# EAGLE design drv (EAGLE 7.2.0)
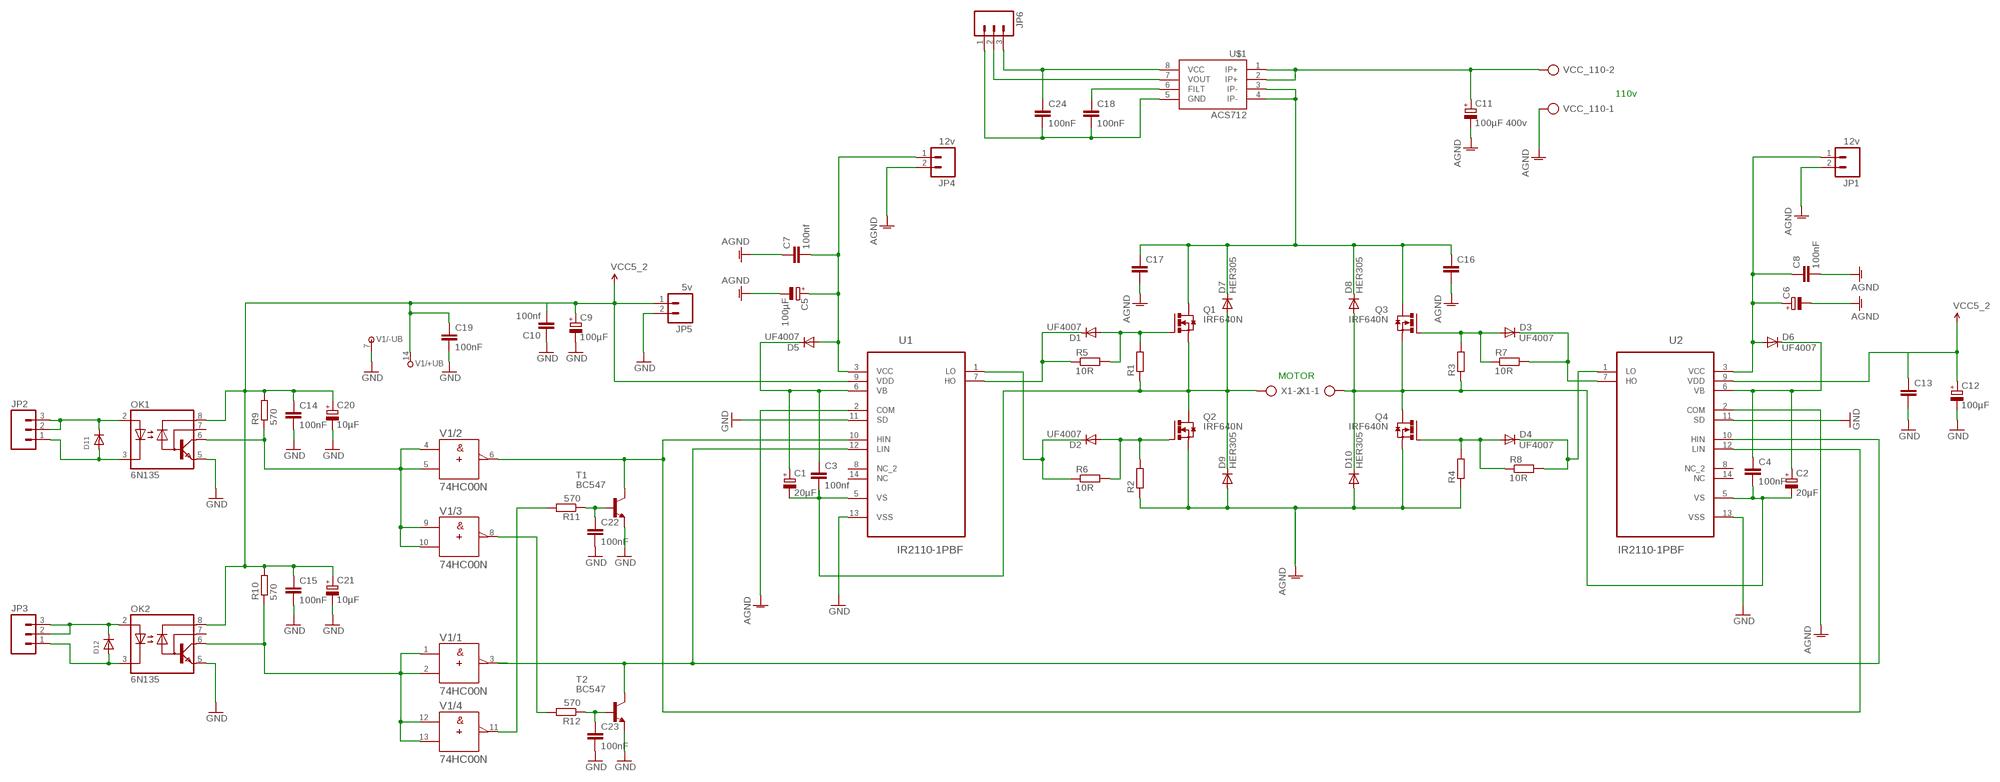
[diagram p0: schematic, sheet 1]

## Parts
C1  20µF  CPOL-EUE2,5-6E  [E2,5-6E]
C2  20µF  CPOL-EUE2,5-6E  [E2,5-6E]
C3  100nf  C-EUC0805  [C0805]
C4  100nF  C-EUC0504  [C0504]
C5  100µF  CPOL-EUE2-5  [E2-5]
C6  CPOL-EUE2-5  [E2-5]
C7  100nf  C-EUC1310  [C1310]
C8  100nF  C-EUC0805  [C0805]
C9  100µF  CPOL-EUE2-5  [E2-5]
C10  100nf  C-EUC0805  [C0805]
C11  100µF 400v  CPOL-EUE10-25  [EB25D]
C12  100µF  CPOL-EUE2-5  [E2-5]
C13  C-EUC0805  [C0805]
C14  100nF  C-EUC0805  [C0805]
C15  100nF  C-EUC0805  [C0805]
C16  C5/3  [C5B3]
C17  C5/3  [C5B3]
C18  100nF  C-EUC0805  [C0805]
C19  100nF  C-EUC0805  [C0805]
C20  10µF  CPOL-EUE2-5  [E2-5]
C21  10µF  CPOL-EUE2-5  [E2-5]
C22  100nF  C-EUC0402  [C0402]
C23  100nF  C-EUC0402  [C0402]
C24  100nF  C-EUC0805  [C0805]
D1  UF4007  DIODE  [DIODE-1N4001-KIT]
D2  UF4007  DIODE  [DIODE-1N4001-KIT]
D3  UF4007  DIODE  [DIODE-1N4001-KIT]
D4  UF4007  DIODE  [DIODE-1N4001-KIT]
D5  UF4007  DIODE  [DIODE-1N4001-KIT]
D6  UF4007  DIODE  [DIODE-1N4001-KIT]
D7  HER305  1N5624  [DO201-15]
D8  HER305  1N5624  [DO201-15]
D9  HER305  1N5624  [DO201-15]
D10  HER305  1N5624  [DO201-15]
D11  DIODEDO-1N4148  [DO-1N4148]
D12  DIODEDO-1N4148  [DO-1N4148]
JP1  12v  M02JST-PTH-VERT  [JST-2-PTH-VERT]
JP2  M03LOCK  [1X03_LOCK]
JP3  M03LOCK  [1X03_LOCK]
JP4  12v  M02JST-PTH-VERT  [JST-2-PTH-VERT]
JP5  5v  M02JST-PTH-VERT  [JST-2-PTH-VERT]
JP6  M03LOCK  [1X03_LOCK]
OK1  6N135  [DIL08]
OK2  6N135  [DIL08]
Q1  IRF640N  IRF3704L-V  [TO262-V]
Q2  IRF640N  IRF3704L-V  [TO262-V]
Q3  IRF640N  IRF3704L-V  [TO262-V]
Q4  IRF640N  IRF3704L-V  [TO262-V]
R1  R-EU_0207/12  [0207/12]
R2  R-EU_0207/12  [0207/12]
R3  R-EU_0207/12  [0207/12]
R4  R-EU_0207/12  [0207/12]
R5  10R  R-EU_0207/12  [0207/12]
R6  10R  R-EU_0207/12  [0207/12]
R7  10R  R-EU_0207/12  [0207/12]
R8  10R  R-EU_0207/12  [0207/12]
R9  570  R-EU_R0805  [R0805]
R10  570  R-EU_R0805  [R0805]
R11  570  R-EU_0204/7  [0204/7]
R12  570  R-EU_0204/7  [0204/7]
T1  BC547  [TO92]
T2  BC547  [TO92]
U1  IR2110-1PBF  [DIP254P762X533-14]
U2  IR2110-1PBF  [DIP254P762X533-14]
U$1  ACS712  [SO08]
V1  74HC00N  [DIL14]
VCC_110  AK300/2  [AK300/2]
X1  AK300/2  [AK300/2]

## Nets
AGND: C5.- C6.- C7.1 C8.2 C11.- C16.2 C17.2 D9.A D10.A JP1.2 JP4.2 Q2.3(S) Q4.3(S) R2.1 R4.1 U1.2(COM) U2.2(COM) VCC_110.1
GND: C9.- C10.1 C12.- C13.2 C14.2 C15.2 C19.2 C20.- C21.- C22.2 C23.2 JP5.2 OK1.5(GND) OK2.5(GND) T1.1(E) T2.1(E) U1.11(SD) U1.13(VSS) U2.11(SD) U2.13(VSS) V1.7(/-UB:-UB)
H_PVR1: C11.+ U$1.1(IP+) U$1.2(IP+) VCC_110.2
N$1: D1.A Q1.1(G) R1.2 R5.2
N$2: C18.1 U$1.6(FILT)
N$3: D11.C JP2.2 JP2.3 OK1.2(A)
N$4: D2.A Q2.1(G) R2.2 R6.2
N$5: D1.C R5.1 U1.7(HO)
N$6: D11.A JP2.1 OK1.3(C)
N$7: D2.C R6.1 U1.1(LO)
N$8: R11.2 V1.11(/4:Y)
N$9: D3.A Q3.1(G) R3.2 R7.1
N$10: D3.C R7.2 U2.7(HO)
N$11: D4.C R8.2 U2.1(LO)
N$12: D12.A JP3.1 OK2.3(C)
N$14: D4.A Q4.1(G) R4.2 R8.1
N$15: C1.+ C3.1 D5.C U1.6(VB)
N$16: T1.3(C) U1.10(HIN) U2.12(LIN) V1.6(/2:Y)
N$17: C2.+ C4.1 D6.C U2.6(VB)
N$18: C18.2 C24.2 JP6.1 U$1.5(GND)
N$19: T2.3(C) U1.12(LIN) U2.10(HIN) V1.3(/1:Y)
N$20: R12.2 V1.8(/3:Y)
N$21: OK1.6(VO) R9.1 V1.4(/2:A) V1.5(/2:B) V1.9(/3:A) V1.10(/3:B)
N$22: C22.1 R11.1 T1.2(B)
N$23: C23.1 R12.1 T2.2(B)
N$24: C24.1 JP6.3 U$1.8(VCC)
N$25: OK2.6(VO) R10.1 V1.1(/1:A) V1.2(/1:B) V1.12(/4:A) V1.13(/4:B)
N$26: D12.C JP3.2 JP3.3 OK2.2(A)
N$28: JP6.2 U$1.7(VOUT)
OUT1: C2.- C4.2 D8.A D10.C Q3.3(S) Q4.2(D) R3.1 U2.5(VS) X1.1
OUT2: C1.- C3.2 D7.A D9.C Q1.3(S) Q2.2(D) R1.1 U1.5(VS) X1.2
VCC: C9.+ C10.2 C12.+ C13.1 C14.1 C15.1 C19.1 C20.+ C21.+ JP5.1 OK1.8(VCC) OK2.8(VCC) R9.2 R10.2 U1.9(VDD) U2.9(VDD) V1.14(/+UB:+UB) ; supply symbol labelled VCC5_2
VCC_12_1: C5.+ C7.2 D5.A JP4.1 U1.3(VCC)
VCC_12_2: C6.+ C8.1 D6.A JP1.1 U2.3(VCC)
VCC_110: C16.1 C17.1 D7.C D8.C Q1.2(D) Q3.2(D) U$1.3(IP-) U$1.4(IP-)
Unconnected: OK1.7(VB) OK2.7(VB) U1.8(NC_2) U1.14(NC) U2.8(NC_2) U2.14(NC)

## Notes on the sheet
- 110v
- MOTOR

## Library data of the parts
C1 C2 C5 C6 C9 C11 C12 C20 C21 = rcl:CPOL-EU: POLARIZED CAPACITOR, European symbol
C3 C4 C7 C8 C10 C13-C15 C18 C19 C22-C24 = rcl:C-EU: CAPACITOR, European symbol
C16 C17 = capacitor-wima:C: CAPACITOR
D1-D6 = SparkFun-DiscreteSemi:DIODE: Diode
D7-D10 = diode:1N5624: DIODE
D11 D12 = adafruit:DIODE: Diode
JP1 JP4 JP5 = SparkFun-Connectors:M02: Standard 2-pin 0.1" header. Use with
JP2 JP3 JP6 = SparkFun-Connectors:M03: Header 3 Standard 3-pin 0.1" header. Use with straight break away headers (SKU : PRT-00116), right angle break away headers (PRT-00553), swiss pins (PRT-00743), machine pins (PRT-00117), and female headers (PRT-00115). Molex polarized connector foot print use with SKU : PRT-08232 with associated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
OK1 OK2 = optocoupler:6N135: MOTOROLA OPTO COUPLER; MF: FAIRCHILD SEMICONDUCTOR; MPN: 6N135; OC_FARNELL: 1021342; OC_NEWARK: 58K9658
Q1-Q4 = transistor-power:IRF3704: SMPS MOSFET HEXFET® Power MOSFET Source: http://www.irf.com/product-info/datasheets/data/irf3704.pdf
R1-R12 = rcl:R-EU_: RESISTOR, European symbol
T1 T2 = transistor:BC547: NPN TRANSISTOR
U1 U2 = International_Rectifier_By_element14_Batch_1:IR2110-1PBF: HIGH AND LOW SIDE DRIVER; MPN: IR2110-1PBF; OC_FARNELL: 1374799; OC_NEWARK: 19K8414; PACKAGE: PDIP-14; SUPPLIER: INTERNATIONAL RECTIFIER
U$1 = SparkFun-AnalogIC:ACS712: Hall-effect-based isolated linear current sensor
V1 = 74ttl-din:74*00: Quad 2-input NAND gate
VCC_110 X1 = con-ptr500:AK300/2: CONNECTOR; OC_FARNELL: unknown; OC_NEWARK: unknown

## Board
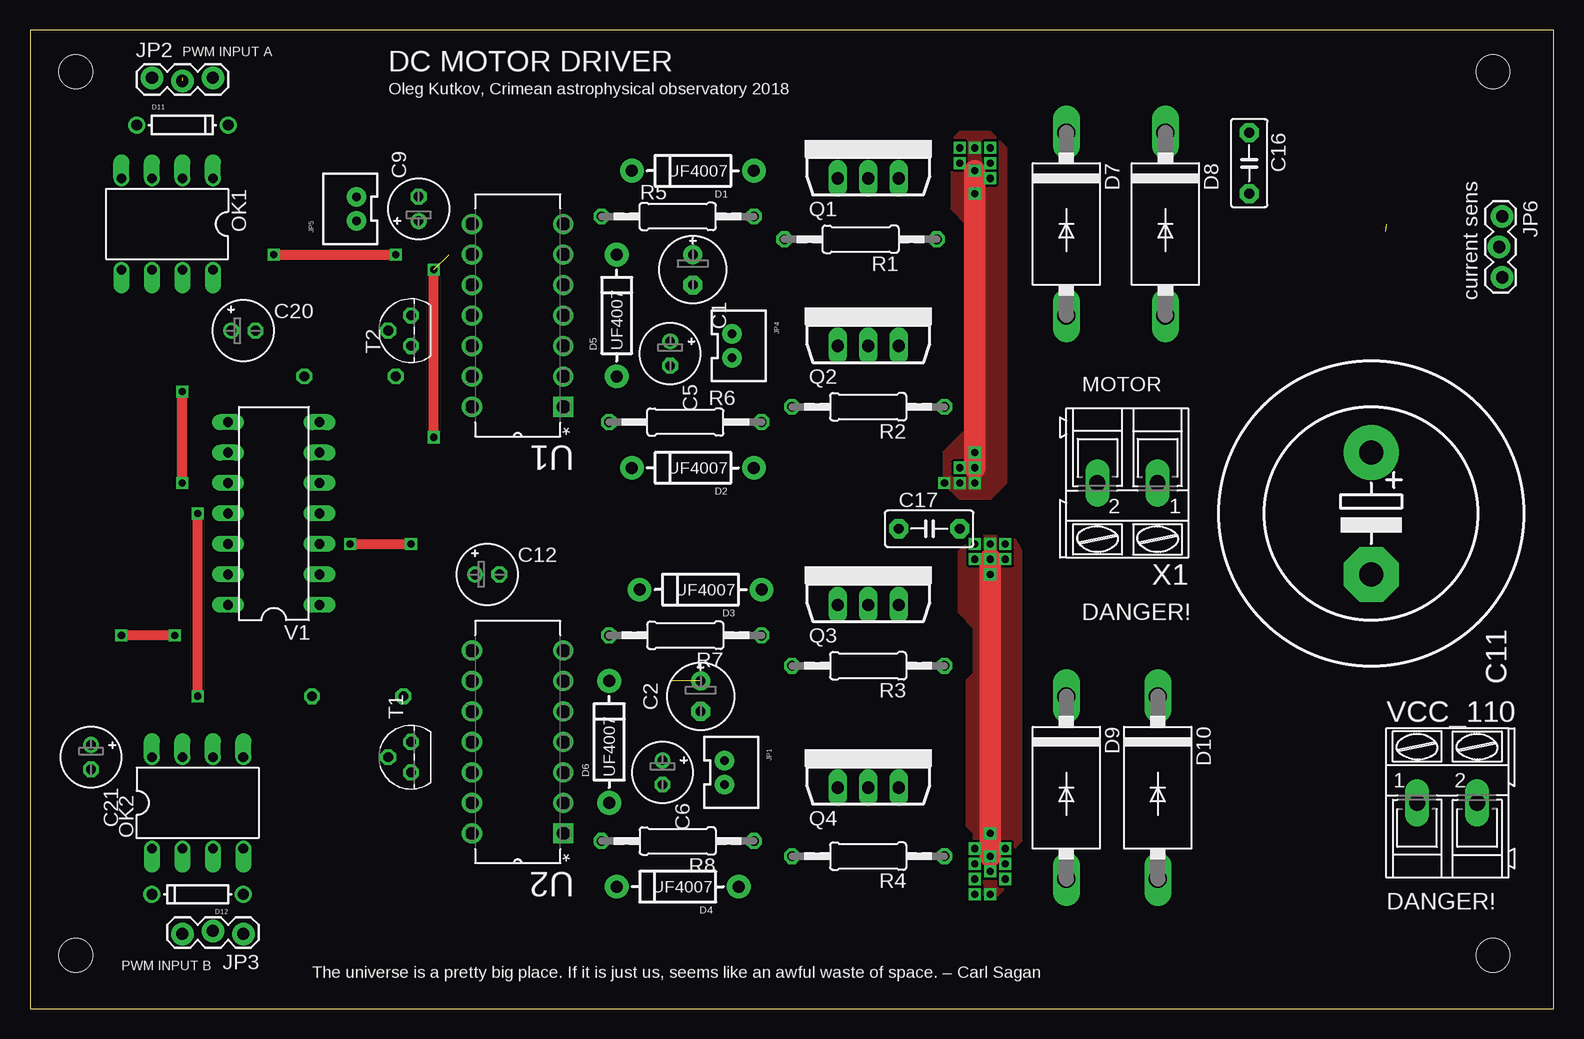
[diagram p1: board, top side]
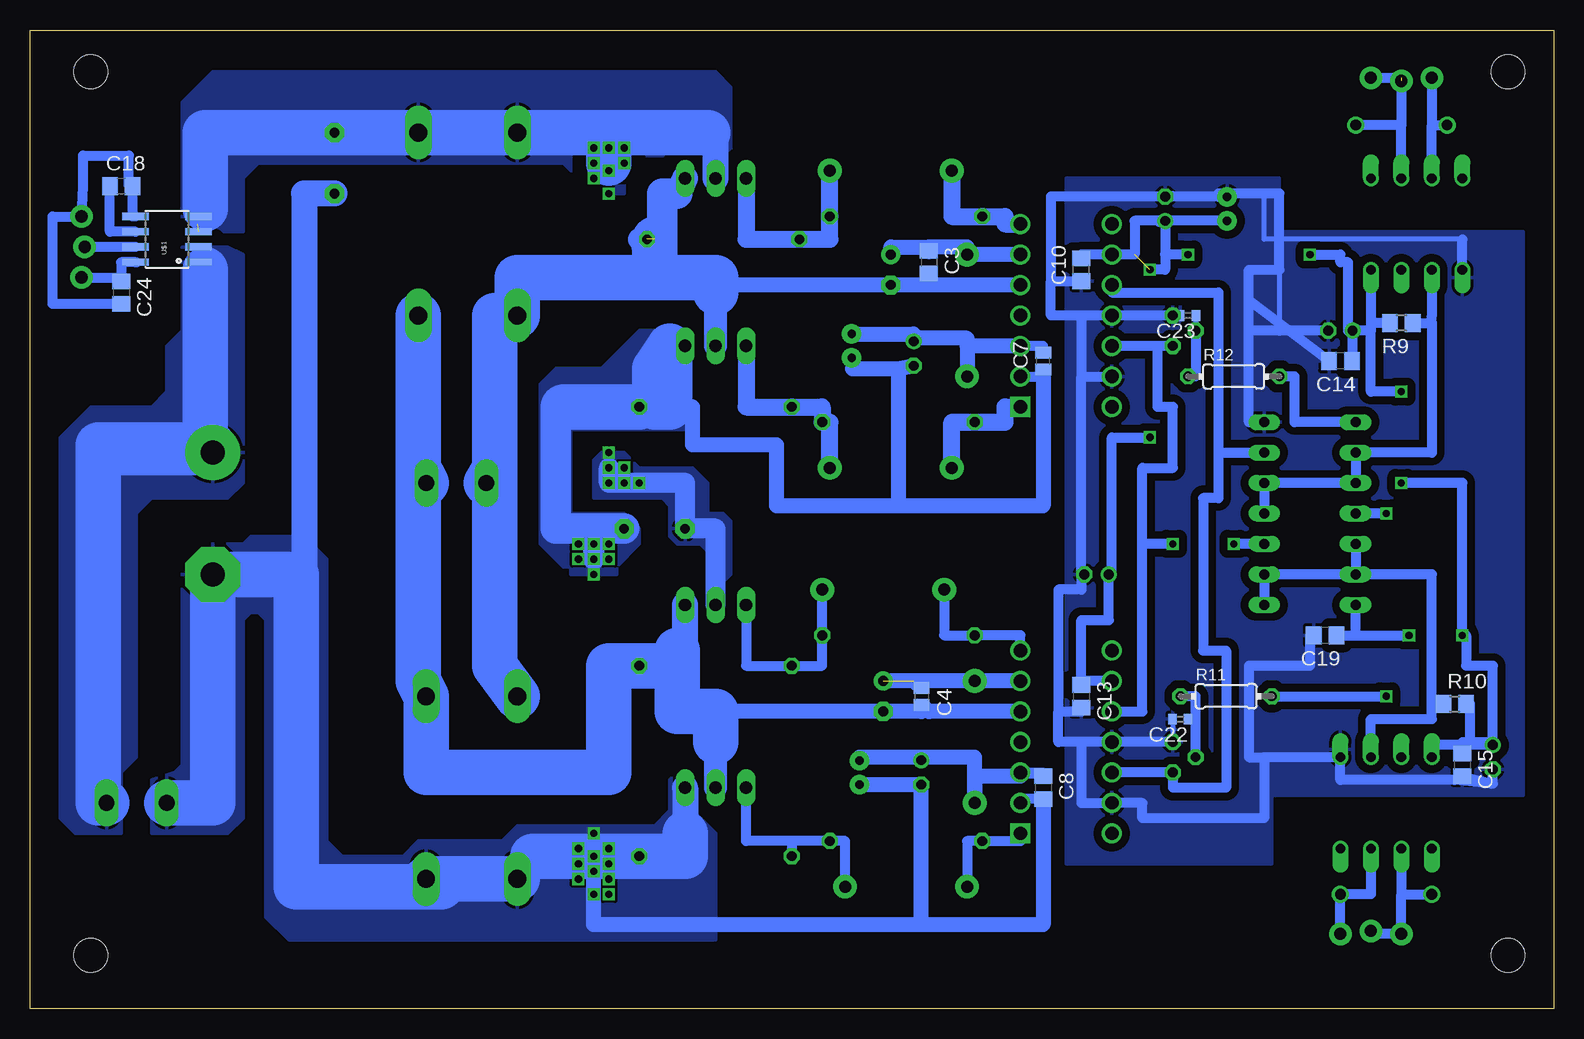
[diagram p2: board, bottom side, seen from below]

Size 126.98 x 81.58 mm. Coordinates in mm from the lower left corner, seen from the top.
Outline: 0,0 126.98,0 126.98,81.58 0,81.58 0,0
Copper layers (1*16): Top 0.035mm / dielectric 1.5mm / Bottom 0.035mm
Design rules "default": minimum track width 10mil, minimum drill 24mil, track to track 8mil, track to pad 8mil, pad to pad 8mil, via to via 8mil, smd to smd 8mil, copper to edge 40mil, drill to drill 8mil, minimum pad ring 10mil, minimum via ring 8mil, stop-mask expansion 4mil, vias tented up to drill 0mil, thermal gap 10mil
Holes 2.8 mm at 3.81,78.11 121.92,78.11 121.92,4.44 3.81,4.44

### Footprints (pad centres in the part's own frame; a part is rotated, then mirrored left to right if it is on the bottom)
E2,5-6E = drill 0.813 pad 1.575: + -1.27,0 | drill 0.813 pad 1.575 octagon: - 1.27,0
C0805 = smd 1.3 x 1.5: 1 -0.95,0; 2 0.95,0
C0504 = smd 1 x 1.3: 1 -0.7,0; 2 0.7,0
E2-5 = drill 0.813 pad 1.27: + -1.016,0 | drill 0.813 pad 1.27 octagon: - 1.016,0
C1310 = smd 1 x 1.3: 1 -0.7,0; 2 0.7,0
EB25D = drill 2.007 pad 4.597: + -5.08,0 | drill 2.007 pad 4.597 octagon: - 5.08,0
C5B3 = drill 0.813 pad 1.6 octagon: 1 -2.54,0; 2 2.54,0
C0402 = smd 0.7 x 0.9: 1 -0.65,0; 2 0.65,0
DIODE-1N4001-KIT = drill 1 pad 1.981: A -5.08,0; C 5.08,0
DO201-15 = drill 1.499 long: A 7.62,0; C -7.62,0
DO-1N4148 = drill 0.9: A -3.81,0; C 3.81,0
JST-2-PTH-VERT = drill 0.7 pad 1.626: 1 -1,-0.55; 2 1,-0.55
1X03_LOCK = drill 1.016 pad 1.88: 1 0,0.127; 2 2.54,-0.127; 3 5.08,0.127
DIL08 = drill 0.813 offset: 1 -3.81,-3.81; 2 -1.27,-3.81; 3 1.27,-3.81; 4 3.81,-3.81; 5 3.81,3.81; 6 1.27,3.81; 7 -1.27,3.81; 8 -3.81,3.81
TO262-V = drill 1.016 long: 1 -2.54,0; 2 0,0; 3 2.54,0
0207/12 = drill 0.813 octagon: 1 -6.35,0; 2 6.35,0
R0805 = smd 1.3 x 1.5: 1 -0.95,0; 2 0.95,0
0204/7 = drill 0.813 octagon: 1 -3.81,0; 2 3.81,0
TO92 = drill 0.813 octagon: 1 1.27,0; 2 0,1.905; 3 -1.27,0
DIP254P762X533-14 = drill 1.118 square: 1 -7.62,15.24 | drill 1.118: 2 -7.62,12.7; 3 -7.62,10.16; 4 -7.62,7.62; 5 -7.62,5.08; 6 -7.62,2.54; 7 -7.62,0; 8 0,0; 9 0,2.54; 10 0,5.08; 11 0,7.62; 12 0,10.16; 13 0,12.7; 14 0,15.24
SO08 = smd 0.61 x 2.21: 1 -1.905,-2.616; 2 -0.635,-2.616; 3 0.635,-2.616; 4 1.905,-2.616; 5 1.905,2.616; 6 0.635,2.616; 7 -0.635,2.616; 8 -1.905,2.616
DIL14 = drill 0.813 long: 1 -7.62,-3.81; 2 -5.08,-3.81; 3 -2.54,-3.81; 4 0,-3.81; 5 2.54,-3.81; 6 5.08,-3.81; 7 7.62,-3.81; 8 7.62,3.81; 9 5.08,3.81; 10 2.54,3.81; 11 0,3.81; 12 -2.54,3.81; 13 -5.08,3.81; 14 -7.62,3.81
AK300/2 = drill 1.321 long: 1 -2.515,0; 2 2.489,0

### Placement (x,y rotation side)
C1  55.24,61.59 270 top
C2  55.88,26.03 270 top
C3  52.07,62.23 270 bottom
C4  52.7,26.03 270 bottom
C5  53.34,54.61 270 top
C6  52.7,19.69 270 top
C7  42.55,53.97 90 bottom
C8  42.55,18.41 270 bottom
C9  32.38,66.67 90 top
C10  39.37,61.59 90 bottom
C11  111.76,41.27 270 top
C12  38.1,36.19 0 top
C13  39.37,26.03 270 bottom
C14  17.78,53.97 180 bottom
C15  7.62,20.32 270 bottom
C16  101.6,70.48 270 top
C17  74.93,40 0 top
C18  119.38,68.58 0 bottom
C19  19.05,31.11 180 bottom
C20  17.78,56.52 0 top
C21  5.08,20.95 270 top
C22  31.11,24.13 180 bottom
C23  30.48,57.78 180 bottom
C24  119.38,59.69 270 bottom
D1  55.24,69.85 180 top
D2  55.24,45.08 180 top
D3  55.88,34.92 180 top
D4  53.98,10.16 180 top
D5  48.9,57.78 90 top
D6  48.26,22.22 90 top
D7  86.36,65.41 270 top
D8  94.61,65.41 270 top
D9  86.36,18.41 270 top
D10  93.98,18.41 270 top
D11  12.7,73.66 0 top
D12  13.97,9.52 180 top
JP1  58.42,19.69 270 top
JP2  10.16,77.47 0 top
JP3  17.78,6.35 180 top
JP4  59.05,55.24 270 top
JP5  26.67,66.67 90 top
JP6  122.56,66.04 270 top
OK1  11.43,65.41 180 top
OK2  13.97,17.14 0 top
Q1  69.85,69.21 0 top
Q2  69.85,55.24 0 top
Q3  69.85,33.66 0 top
Q4  69.85,18.41 0 top
R1  69.22,64.13 180 top
R2  69.85,50.16 180 top
R3  69.85,28.58 180 top
R4  69.85,12.7 180 top
R5  53.98,66.04 0 top
R6  54.61,48.89 0 top
R7  54.61,31.11 180 top
R8  53.98,13.97 180 top
R9  12.7,57.15 180 bottom
R10  8.26,25.4 0 bottom
R11  27.3,26.03 0 bottom
R12  26.67,52.7 0 bottom
T1  31.75,20.95 90 top
T2  31.75,56.52 90 top
U1  36.83,65.41 180 top
U2  36.83,29.84 180 top
U$1  115.57,64.13 90 bottom
V1  20.32,41.27 90 top
VCC_110  118.11,17.14 0 top
X1  91.44,43.81 180 top

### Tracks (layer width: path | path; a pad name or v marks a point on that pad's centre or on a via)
AGND  (via drill 0.6)
  Top 1.778: v80.01,37.47 v80.01,36.19 v80.01,14.61 v80.01,12.7
  Bottom 0.406: C7.1 42.55,52.7
  Bottom 0.813: C6.- 56.6,18.67 JP1.2 | C8.2 44.45,17.47 U2.2 | U1.2 42.55,52.7
  Bottom 1.27: C8.2 42.55,6.98 52.7,6.98 | 52.7,6.98 C6.- 52.7,18.69 JP1.2 | 52.7,6.98 80.01,6.98 v80.01,9.52 80.01,12.06 | 42.55,52.7 42.55,41.91 54.61,41.91 | 54.61,53.34 C5.- | JP4.2 58.42,54.24 58.42,53.34 54.61,53.34 | 54.61,53.34 54.61,41.91 | 54.61,41.91 64.77,41.91 64.77,46.99 71.75,46.99 71.75,50.16 74.93,50.16 R2.1 | Q2.3 73.66,55.24
  Bottom 1.778: 85.09,12.7 D9.A | v80.01,37.47 v80.01,38.73 80.01,40 83.19,40
  Bottom 2.184: C16.2 104.14,67.95 104.14,36.19 C11.- | Q4.3 72.39,14.61
  Bottom 2.54: C17.2 83.19,40 83.19,50.16 82.55,50.16
  Bottom 3.81: D9.A D10.A 92.71,10.16 104.78,10.16 104.78,36.19 C11.- 111.76,17.14 VCC_110.1 | 85.09,12.7 v80.01,12.7 R4.1 72.39,12.7 72.39,14.61 | 74.93,51.44 74.93,53.34 73.66,55.24 73.66,50.16 74.93,50.16 | R2.1 82.55,50.16
  pour Bottom: 116.84,19.05 116.84,14.61 110.49,14.61 109.22,15.88 109.22,32.38 108.58,33.02 107.95,33.02 107.31,32.38 107.31,7.62 105.41,5.72 69.85,5.72 69.85,14.61 71.75,16.51 71.75,19.69 73.03,19.69 73.66,19.05 73.66,16.51 74.93,15.24 86.36,15.24 87.63,13.97 94.61,13.97 95.89,12.7 100.97,12.7 102.23,13.97 102.23,37.47 104.14,39.37 108.58,39.37 109.22,38.73 112.39,38.73 114.3,36.83 114.3,20.32 114.94,19.69
  pour Top: 77.47,33.02 77.47,38.1 78.74,39.37 81.92,39.37 82.55,38.1 82.55,13.97 81.92,13.33 81.92,10.8 80.64,9.52 79.38,9.52 78.74,10.16 78.74,14.61 78.11,15.24 78.11,27.3 78.74,27.94 78.74,31.75
  pour Bottom: 76.2,40 76.2,38.73 78.11,36.83 78.11,36.19 81.92,36.19 81.92,36.83 82.55,36.83 84.45,38.73 84.45,52.07 83.19,53.34 79.38,53.34 76.2,56.52 72.39,56.52 72.39,48.26 81.92,48.26 81.92,41.27 77.47,41.27 76.83,40.64
GND
  Bottom 0.406: C9.- 32.38,67.95 31.75,67.95 | C23.2 T2.1 | C22.2 T1.1 | 7.62,64.13 24.13,64.13 24.13,67.95 | 22.86,67.95 22.86,56.52
  Bottom 0.813: JP5.2 27.94,67.67 | 27.94,67.67 32.38,67.67 C9.- 41.91,67.69 41.91,60.64 | 41.91,60.64 C10.1 | 39.37,57.78 U1.11 T2.1 | 39.37,57.78 39.37,52.7 | 39.37,52.7 U1.13 | 39.37,36.19 39.37,52.7 | C12.- 39.37,36.19 | 39.37,36.19 39.37,34.92 41.27,34.92 41.27,24.77 | 41.27,24.77 39.37,24.77 C13.2 | 39.37,22.22 U2.11 T1.1 | 39.37,22.22 39.37,17.14 U2.13 34.29,17.14 34.29,15.88 24.13,15.88 24.13,20.95 | 39.37,22.22 41.27,22.22 41.27,24.77 | 39.37,57.78 41.91,57.78 41.91,60.64 | 27.94,67.67 27.94,67.95 24.13,67.95 22.86,67.95 22.86,61.59 25.4,61.59 25.4,59.05 | V1.7 25.4,48.89 25.4,56.52 | 25.4,56.52 25.4,59.05 | C19.2 20.32,31.11 20.32,28.58 25.4,28.58 25.4,20.95 24.13,20.95 | 24.13,20.95 OK2.5 17.78,19.05 8.26,19.05 5.08,18.73 | C20.- 19.05,56.52 22.86,56.52 25.4,56.52 | C14.2 25.4,59.05 | C15.2 5.08,18.73 | 5.08,18.73 C21.- | OK1.5 7.62,64.13
  pour Bottom (isolate 0.66): 2.54,64.77 22.86,64.77 22.86,69.21 40.64,69.21 40.64,12.06 23.5,12.06 23.5,17.78 2.54,17.78
H_PVR1
  Bottom 0.305: U$1.2 U$1.1 112.39,62.23 112.39,61.59
  Bottom 3.81: 121.28,46.36 121.28,46.99 112.39,46.99 | VCC_110.2 121.28,17.14 121.28,46.36 | 121.28,46.36 C11.+ 111.76,46.99 112.39,46.99 | 112.39,46.99 112.39,61.59
  pour Bottom (isolate 0.813): 114.3,63.5 110.49,63.5 109.22,62.86 109.22,43.81 110.49,42.55 116.84,42.55 118.11,41.27 118.11,20.95 119.38,19.69 119.38,14.61 123.19,14.61 124.46,15.88 124.46,47.62 121.92,50.16 116.84,50.16 115.57,51.44 115.57,55.24 114.3,56.52
N$1
  Bottom 1.422: Q1.1 67.31,64.13 R1.2 60.33,64.13 R5.2 D1.A
N$2
  Bottom 0.813: U$1.6 120.33,64.77 C18.1
N$3  (1 unrouted)
  Bottom 0.813: OK1.2 12.7,73.66 | 12.7,73.66 D11.C | JP2.3 12.7,77.6 12.7,73.66
N$4
  Bottom 1.422: Q2.1 67.31,50.16 R2.2 60.96,50.16 R6.2 60.33,48.89 D2.A
N$5
  Bottom 1.422: D1.C 50.16,66.04 R5.1 45.72,66.04 45.72,65.41 U1.7
N$6
  Bottom 0.813: OK1.3 10.16,73.66 | 10.16,73.66 D11.A | JP2.1 10.16,73.66
N$7
  Bottom 1.422: D2.C 50.16,48.89 R6.1 45.72,48.89 45.72,50.16 U1.1
N$8  (via drill 0.6)
  Top 0.813: v13.97,26.03 v13.97,41.27
  Bottom 0.813: R11.2 v13.97,26.03 | v13.97,41.27 V1.11
N$9
  Bottom 0.813: D3.A R7.1 60.96,28.58 R3.2 67.31,28.58 Q3.1
N$10
  Bottom 0.813: D3.C 50.8,31.11 R7.2 44.45,31.11 U2.7
N$11
  Bottom 0.813: U2.1 44.45,13.97 R8.2 48.9,13.97 D4.C
N$12
  Bottom 0.813: OK2.3 15.24,9.52 D12.A JP3.1
N$13  (via drill 0.6)
  other vias: 77.47,45.08
N$14
  Bottom 0.813: 63.5,13.97 R8.1 59.05,13.97 D4.A | 63.5,13.97 R4.2 | 63.5,13.97 67.31,13.97 Q4.1
N$15
  Bottom 0.813: 52.07,62.86 C3.1 | 55.24,63.18 C1.+
  Bottom 1.27: U1.6 D5.C 48.9,63.5 52.07,63.5 | C1.+ 55.24,63.5 52.07,63.5 | 52.07,63.5 C3.1
N$16
  Bottom 0.61: 36.83,59.69 U1.10
  Bottom 0.813: 36.83,59.69 27.94,59.69 27.94,46.36 | 27.94,46.36 V1.6 | U2.12 T1.3 31.75,18.41 27.3,18.41 27.3,29.84 29.21,29.84 29.21,42.55 27.94,42.55 27.94,46.36
N$17  (1 unrouted)
  Bottom 0.406: C4.1 53.34,26.73 53.34,27.3
  Bottom 0.813: 52.7,27.3 C4.1
  Bottom 1.27: U2.6 D6.C C2.+
N$18
  Bottom 0.813: U$1.5 118.43,66.04 C18.2 118.75,68.58 118.75,71.12 122.56,71.12 122.56,68.58 JP6.1 125.09,66.04 125.09,58.74 C24.2
N$19  (via drill 0.6)
  Top 0.813: v26.67,38.73 v31.75,38.73
  Bottom 0.813: T2.3 33.02,55.24 | 33.02,55.24 U1.12 | U2.10 34.29,24.77 34.29,38.73 | 34.29,38.73 34.29,45.08 31.75,45.08 31.75,50.16 33.02,50.16 33.02,55.24 | V1.3 v26.67,38.73 | v31.75,38.73 34.29,38.73
N$20
  Bottom 0.813: V1.8 21.59,48.89 21.59,52.7 R12.2
N$21
  Bottom 0.813: V1.4 V1.5 V1.10 V1.9 10.16,46.36 10.16,57.15 | OK1.6 10.16,57.78 10.16,57.15 | R9.1 10.16,57.15
N$22
  Bottom 0.406: C22.1 29.84,24.13 29.84,24.77
  Bottom 0.813: T1.2 29.84,24.77 29.84,26.03 R11.1
N$23
  Bottom 0.406: C23.1 29.84,57.15 T2.2
  Bottom 0.813: T2.2 29.84,52.7 R12.1
N$24
  Bottom 0.813: 118.11,62.23 U$1.8 119.38,62.23 C24.1 119.38,60.96 JP6.3
N$25
  Bottom 0.813: V1.12 V1.13 | V1.13 V1.2 V1.1 | OK2.6 15.24,24.13 10.16,24.13 10.16,25.4 | 10.16,25.4 10.16,36.19 V1.13 | R10.1 10.16,25.4
N$26
  Bottom 0.813: OK2.2 12.7,9.52 | 12.7,9.52 D12.C | JP3.2 15.24,6.22 JP3.3 12.7,9.52
N$27  (via drill 0.6)
  other vias: 80.01,11.43
N$28
  Bottom 0.813: U$1.7 JP6.2
N$29  (via drill 0.6)
  other vias: 81.28,38.73
N$30  (via drill 0.6)
  other vias: 81.28,37.47
N$31  (via drill 0.6)
  other vias: 78.74,38.73
N$32  (via drill 0.6)
  other vias: 78.74,37.47
N$33  (via drill 0.6)
  other vias: 80.01,71.76
N$34  (via drill 0.6)
  other vias: 80.01,70.48
N$35  (via drill 0.6)
  other vias: 80.01,69.21
N$36  (via drill 0.6)
  other vias: 77.47,70.48
N$37  (via drill 0.6)
  other vias: 77.47,71.76
N$38  (via drill 0.6)
  other vias: 81.28,12.06
N$39  (via drill 0.6)
  other vias: 81.28,10.8
N$40  (via drill 0.6)
  other vias: 78.74,9.52
N$41  (via drill 0.6)
  other vias: 78.74,10.8
N$42  (via drill 0.6)
  other vias: 78.74,12.06
N$43  (via drill 0.6)
  other vias: 78.74,13.33
N$44  (via drill 0.6)
  other vias: 81.28,13.33
OUT1
  Bottom 0.406: 52.07,24.77 52.7,24.77 C4.2 52.07,25.33 52.07,24.77
  Bottom 1.27: U2.5 52.07,24.77 | 52.7,24.77 C2.- 69.85,24.77
  Bottom 1.778: D10.C 93.95,26.03
  Bottom 1.93: Q4.2 69.85,22.22
  Bottom 2.184: 73.03,29.84 72.39,29.84 Q3.3
  Bottom 3.81: 73.03,28.58 R3.1 78.74,28.58 78.74,19.69 93.98,19.69 D10.C 94.61,27.3 | 73.03,28.58 73.03,29.84 | 93.95,26.03 94.61,27.3 | 73.03,28.58 73.03,24.77 69.85,24.77 69.85,22.22 | D8.A 94.61,45.08 | 94.61,45.08 94.59,45.08 X1.1 94.61,45.08 | 94.61,45.08 94.61,27.3
OUT2  (1 unrouted)
  Bottom 0.406: C3.2 52.07,60.33
  Bottom 1.27: U1.5 52.07,60.33 C1.- 69.85,60.33
  Bottom 1.93: R1.1 76.2,64.13 | Q2.2 69.85,59.69 69.85,60.33
  Bottom 2.184: Q1.3 73.03,67.95
  Bottom 2.54: 73.03,67.95 74.3,67.95 74.3,63.5 75.56,63.5 R1.1
  Bottom 3.81: D9.C 88.27,28.58 88.27,45.08 | X1.2 88.27,45.08 | 88.27,45.08 88.27,57.78 D7.A 86.36,60.96 74.93,60.96 | 69.85,59.69 69.85,60.96 74.93,60.96 | 74.93,60.96 74.93,64.13
VCC  (via drill 0.6)  (1 unrouted)
  Top 0.813: v33.66,47.62 v33.66,61.59 | v20.32,62.86 v30.48,62.86 | v12.06,31.11 v7.62,31.11 | v12.7,43.81 v12.7,51.44
  Bottom 0.406: 39.37,27.3 C13.1 | C9.+ 32.38,65.41 33.02,65.41 33.02,65.67
  Bottom 0.813: 27.22,65.41 JP5.1 34.92,65.67 34.92,62.86 U1.9 39.37,62.86 C10.2 | C9.+ 32.38,62.86 | 32.38,62.86 32.38,61.59 v33.66,61.59 | v33.66,47.62 36.83,47.62 36.83,36.19 C12.+ 37.08,32.38 39.37,32.38 39.37,27.3 U2.9 | C19.1 16.51,31.11 | 16.51,31.11 V1.14 | v30.48,62.86 32.38,62.86 | 16.51,31.11 v12.06,31.11 | OK2.8 10.16,21.97 C21.+ 5.08,22.22 | C15.1 7.62,22.22 6.99,22.22 | 6.99,22.22 5.08,22.22 | 5.08,22.22 5.08,28.58 7.3,28.58 7.3,31.11 v7.62,31.11 7.62,43.81 v12.7,43.81 | v12.7,51.44 15.24,51.44 15.24,56.52 | 15.24,56.52 C20.+ | v20.32,62.86 17.78,62.86 17.78,62.23 17.14,62.23 17.14,56.52 C20.+ | 15.49,61.59 OK1.8 15.24,57.15 | C14.1 16.76,53.97 C20.+ | R10.2 6.99,25.4 6.99,22.22 | R9.2 15.24,57.15 | 15.24,57.15 15.24,56.52
VCC_12_1
  Bottom 0.813: C7.2 42.55,55.24 U1.3
  Bottom 1.27: U1.3 48.9,55.24 | 48.9,55.24 D5.A | 48.9,55.24 48.9,55.88 53.34,55.88 C5.+ 53.34,56.24 JP4.1
VCC_12_2
  Bottom 0.406: C8.1 44.45,19.36 U2.3
  Bottom 0.813: U2.3 42.55,19.69
  Bottom 1.27: 44.45,19.36 48.26,19.36 D6.A 48.26,20.95 52.7,20.95 | C6.+ 52.7,20.95 | 52.7,20.95 57.87,20.95 JP1.1
VCC_110  (via drill 0.6)  (1 unrouted)
  Top 1.778: v78.74,69.85 v78.74,67.95 v78.74,46.36 v78.74,45.08
  Bottom 0.305: U$1.4 113.03,65.41 112.39,66.67
  Bottom 0.813: D8.C 72.39,73.02 69.85,73.02
  Bottom 1.676: Q3.2 69.85,40 C17.1 72.39,43.81 v76.2,43.81 v77.47,43.81 v78.74,43.81 v78.74,45.08
  Bottom 2.184: 78.74,73.02 v78.74,71.76 78.74,70.48 v78.74,69.85 | Q1.2 69.85,73.02
  Bottom 3.81: 78.74,73.02 D7.C D8.C C16.1 112.39,73.02 112.39,66.67 | 70.48,73.02 72.39,73.02 78.74,73.02 | 78.74,73.02 78.74,70.48
  pour Bottom (isolate 1.27): 68.58,67.95 68.58,76.83 69.85,78.11 111.76,78.11 114.3,75.56 114.3,64.77 109.22,64.77 109.22,69.21 107.95,70.48 82.55,70.48 80.01,67.95 77.47,67.95 77.47,70.48 76.83,71.12 71.75,71.12 71.12,70.48 71.12,67.95
  pour Top: 77.47,73.02 80.01,73.02 81.28,71.76 81.28,43.81 80.01,42.55 77.47,42.55 76.2,43.81 76.2,46.36 78.11,48.26 78.11,65.41 76.83,66.67 76.83,72.39
  pour Bottom: 69.22,34.92 69.22,33.02 70.48,33.02 70.48,35.56
  pour Bottom: 78.74,46.36 77.47,46.36 76.2,45.08 71.75,45.08 70.48,43.81 70.48,41.27 69.22,41.27 68.58,40.64 68.58,36.19 69.22,35.56 69.22,32.38 70.48,32.38 70.48,38.1 71.12,38.73 73.03,38.73 73.66,39.37 73.66,41.91 74.3,42.55 80.01,42.55 80.01,45.72 79.38,46.36

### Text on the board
tNames: PWM INPUT A | DC MOTOR DRIVER | Oleg Kutkov, Crimean astrophysical observatory 2018 | current sens | MOTOR | DANGER! | DANGER! | PWM INPUT B | The universe is a pretty big place. If it is just us, seems like an awful waste of space. – Carl Sagan

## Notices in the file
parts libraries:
SparkFun-DiscreteSemi: Licensing: Creative Commons ShareAlike 4.0 International - https://creativecommons.org/licenses/by-sa/4.0
